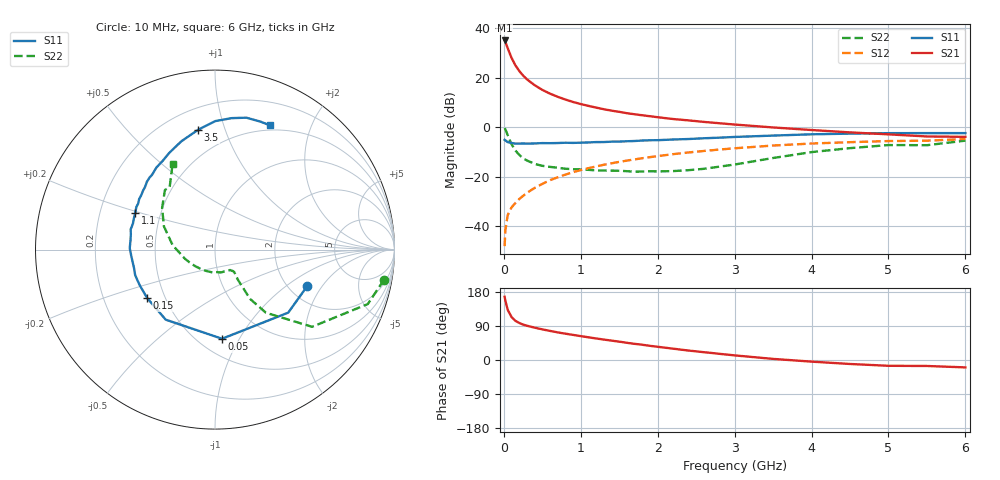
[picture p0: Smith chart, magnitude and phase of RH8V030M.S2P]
! SIEMENS Small Signal Semiconductors
! BFR106
! Si NPN RF Bipolar Junction Transistor in SOT23
! VCE = 8 V  IC = 30 mA
! Common Emitter S-Parameters:  August  1996
# GHz  S  MA  R  50
!  f  S11  S21  S12  S22
! GHz  MAG  ANG  MAG  ANG  MAG  ANG  MAG  ANG
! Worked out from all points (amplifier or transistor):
!   36 points, 10 MHz to 6 GHz, reference 50 ohm
!   highest |S21| = 35.1 dB at 10 MHz (marker M1)
!   |S21| within 3 dB of that: start of sweep to 48.69 MHz
!   unconditionally stable (mu >= 1): 324.9 MHz to 2.155 GHz
!   at 250 MHz: K = 0.94, MSG = 24.4 dB, |S12| = -27.8 dB
!   at 1.4 GHz: K = 1.06, MAG = 9.1 dB, |S12| = -14.6 dB
!   at 6 GHz: K = 0.98, MSG = 0.5 dB, |S12| = -4.8 dB
!   S11 on the Smith chart (normalised r, x): 10 MHz: 2.51, -1.46; 50 MHz: 0.64, -0.85; 150 MHz: 0.40, -0.28; 1.1 GHz: 0.36, +0.19; 3.5 GHz: 0.33, +0.81; 6 GHz: 0.45, +1.44
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0.01  0.5528 -21.5  56.73 166.8  0.0039 82.4  0.9569 -10.1
0.02  0.5384 -40.7  53.03 156.6  0.0083 74.0  0.9039 -19.6
0.05  0.4982 -85.5  39.66 132.6  0.0165 60.2  0.691 -38.5
0.1  0.4773 -125.1  25.21 113.5  0.0237 56.4  0.4521 -51.1
0.15  0.4645 -144.3  17.81 103.4  0.0292 58.6  0.3365 -54.6
0.2  0.4641 -154.8  13.73 97.8  0.0351 61.2  0.2759 -53.9
0.25  0.467 -162.2  11.07 93.4  0.0406 63.1  0.2333 -53.3
0.3  0.4627 -167.4  9.291 90.4  0.0468 65.7  0.2114 -52.8
0.4  0.4675 -175.3  7.062 85.4  0.0588 67.5  0.1805 -50.7
0.5  0.4751 179.1  5.669 80.8  0.0709 68.7  0.1648 -49.4
0.6  0.4735 174.0  4.763 76.8  0.0843 68.8  0.1569 -49.9
0.7  0.4766 169.7  4.11 72.9  0.0966 68.9  0.1506 -51.4
0.9  0.4796 162.5  3.229 66.2  0.1225 67.8  0.1409 -53.9
1.1  0.4896 155.1  2.69 59.9  0.1475 66.2  0.1366 -60.8
1.3  0.4989 149.2  2.304 53.9  0.1732 64.1  0.132 -67.3
1.6  0.5179 140.8  1.913 45.4  0.2102 60.6  0.1283 -80.6
2.2  0.5619 125.5  1.459 29.9  0.2839 52.9  0.129 -113.5
2.8  0.6117 111.4  1.199 16.4  0.3513 44.3  0.1584 -153.1
3.5  0.6743 98.0  0.985 2.9  0.4241 34.2  0.2374 174.0
4.5  0.7383 82.8  0.783 -10.5  0.4963 19.1  0.3756 141.7
5.5  0.7567 70.3  0.647 -15.8  0.5323 8.6  0.4306 125.9
6  0.7568 66.1  0.636 -19.5  0.5731 1.2  0.5327 116.3
